{attribute 'GUID' := '56AA2C34-D736-E752-6308-29B40FF3D0B1'}
TYPE DUT_BalluffSmartLightIn :
STRUCT
		 {attribute 'GUID' := '18071995-0000-0000-0000-000000000010}
		ErrorBit0 : BIT;
		 {attribute 'GUID' := '18071995-0000-0000-0000-000000000010}
		ErrorBit1 : BIT;
		 {attribute 'GUID' := '18071995-0000-0000-0000-000000000010}
		ErrorBit2 : BIT;
		 {attribute 'hide'}
		_reserved1 : BIT;
		 {attribute 'hide'}
		_reserved2 : BIT;
		 {attribute 'hide'}
		_reserved3 : BIT;
		 {attribute 'hide'}
		_reserved4 : BIT;
		 {attribute 'hide'}
		_reserved5 : BIT;
END_STRUCT
END_TYPE
